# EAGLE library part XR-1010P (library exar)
Second order switched capacitor FILTER
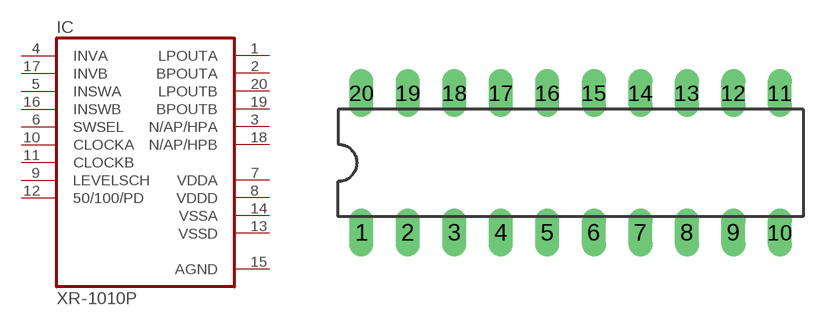
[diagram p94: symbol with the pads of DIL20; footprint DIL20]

Designator prefix IC

## XR-1010P (OC_FARNELL: unknown; OC_NEWARK: unknown)  [DIL20]
1  LPOUTA  out
2  BPOUTA  out
3  N/AP/HPA  out
4  INVA  in
5  INSWA  in
6  SWSEL  in
7  VDDA  pwr
8  VDDD  pwr
9  LEVELSCH  in
10  CLOCKA  in
11  CLOCKB  in
12  50/100/PD  in
13  VSSD  pwr
14  VSSA  pwr
15  AGND  pwr
16  INSWB  in
17  INVB  in
18  N/AP/HPB  out
19  BPOUTB  out
20  LPOUTB  out

## Footprint DIL20 (pad centres in mm)
Dual In Line Package
drill 0.813 long: 1 -11.43,-3.81; 2 -8.89,-3.81; 3 -6.35,-3.81; 4 -3.81,-3.81; 5 -1.27,-3.81; 6 1.27,-3.81; 7 3.81,-3.81; 8 6.35,-3.81; 9 8.89,-3.81; 10 11.43,-3.81; 11 11.43,3.81; 12 8.89,3.81; 13 6.35,3.81; 14 3.81,3.81; 15 1.27,3.81; 16 -1.27,3.81; 17 -3.81,3.81; 18 -6.35,3.81; 19 -8.89,3.81; 20 -11.43,3.81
